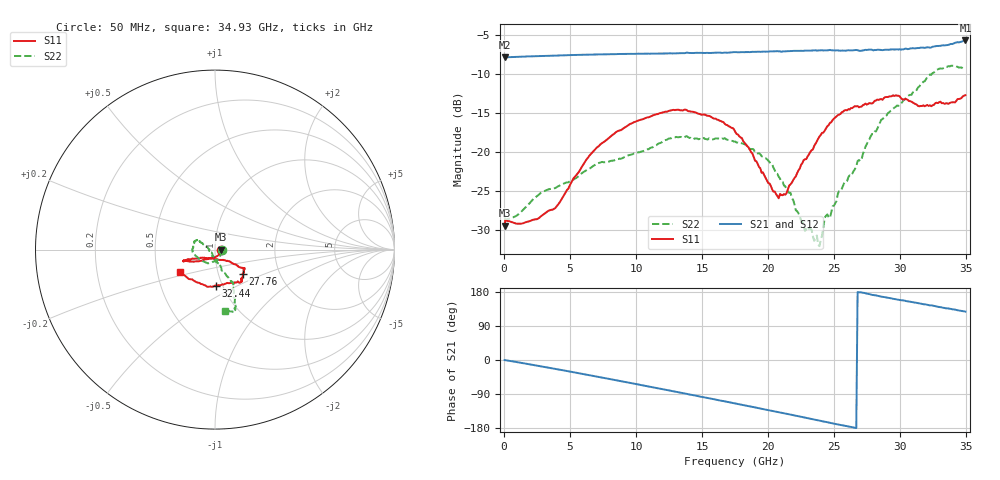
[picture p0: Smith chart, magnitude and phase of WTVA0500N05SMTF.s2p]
! 50 ohm 2-Port S-parameters measured by Modelithics Inc support@modelithics.com  Tampa, FL USA 813-866-6335 (February 2024)
! Smiths Interconnect,  5dB P/N: WTVA0500N05SMTF, Temperature: -50 C
! Board: 10 mil Rogers 4350B, Mounting Pad Dimensions: Length: 15 mils, Width: 25 mils, Gap: 40 mils.
# Hz S RI R 50
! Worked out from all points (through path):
!   352 points, 50 MHz to 34.93 GHz, reference 50 ohm
!   highest |S21| = -5.65 dB at 34.93 GHz (marker M1); lowest = -7.8 dB at 50 MHz (marker M2)
!   group delay of S21, straight-line fit = 18.9 ps
!   lowest |S11| = -29.4 dB at 50 MHz (marker M3), VSWR 1.07, Z = 53.5 - j0.0864 ohm
!   |S11| at or under -10 dB: start of sweep to end of sweep
!   |S22| runs from -32.0 to -8.9 dB; largest |S21 - S12| = 0.0029
!   S11 on the Smith chart (normalised r, x): 50 MHz: 1.07, -0.00; 27.76 GHz: 1.31, -0.37; 32.44 GHz: 0.93, -0.39; 34.93 GHz: 0.65, -0.17
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5e7  0.0339 -0.000806  0.4067 -0.00134  0.4067 -0.00158  0.0383 -0.000766
3.8815e9  -0.00839 -0.0431  0.383 -0.1658  0.3827 -0.166  0.0133 -0.0575
5.8715e9  -0.0577 -0.0556  0.3408 -0.2496  0.3406 -0.2496  -0.0179 -0.071
8.4585e9  -0.1164 -0.0671  0.2553 -0.3415  0.255 -0.3415  -0.0568 -0.0697
1.1742e10  -0.1667 -0.062  0.1097 -0.4161  0.1091 -0.4161  -0.1096 -0.0329
1.3732e10  -0.1764 -0.0653  0.0112 -0.4334  0.011 -0.4332  -0.1262 -0.0026
1.7513e10  -0.1256 -0.0497  -0.1841 -0.3994  -0.1844 -0.3991  -0.105 0.0524
1.9901e10  -0.0465 -0.0467  -0.2935 -0.3313  -0.2933 -0.3314  -0.0804 0.0414
2.07965e10  -0.00822 -0.0501  -0.3309 -0.2968  -0.3311 -0.2964  -0.0639 0.028
2.1692e10  0.0228 -0.0582  -0.3618 -0.2615  -0.3618 -0.2612  -0.0524 0.0169
2.27865e10  0.0637 -0.0639  -0.3966 -0.2113  -0.3966 -0.2109  -0.0314 0.000794
2.33835e10  0.0813 -0.0656  -0.4113 -0.1812  -0.4112 -0.1808  -0.0285 -0.00519
2.3682e10  0.0914 -0.0737  -0.4185 -0.164  -0.4183 -0.1638  -0.0247 -0.0158
2.3881e10  0.0998 -0.0776  -0.4235 -0.1554  -0.4234 -0.1553  -0.0171 -0.0183
2.4279e10  0.1111 -0.0816  -0.4302 -0.1334  -0.4302 -0.1331  -0.0155 -0.0349
2.4677e10  0.1263 -0.0893  -0.4401 -0.1119  -0.44 -0.112  -0.00815 -0.0371
2.53735e10  0.1436 -0.1  -0.4445 -0.0715  -0.4443 -0.0717  0.00131 -0.0565
2.7065e10  0.1602 -0.1137  -0.4488 0.0131  -0.4486 0.0133  0.0253 -0.0864
2.77615e10  0.1547 -0.1366  -0.4529 0.0571  -0.4527 0.0574  0.0396 -0.1208
2.91545e10  0.1464 -0.1753  -0.4365 0.1277  -0.4363 0.1279  0.08 -0.1622
3.2438e10  0.00339 -0.2003  -0.3835 0.2814  -0.3829 0.2821  0.1118 -0.3018
3.49255e10  -0.1961 -0.1251  -0.3194 0.413  -0.3179 0.4139  0.0537 -0.3394
